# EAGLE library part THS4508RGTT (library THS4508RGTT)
Wideband Fully Differential Amplifier Source: Datasheet
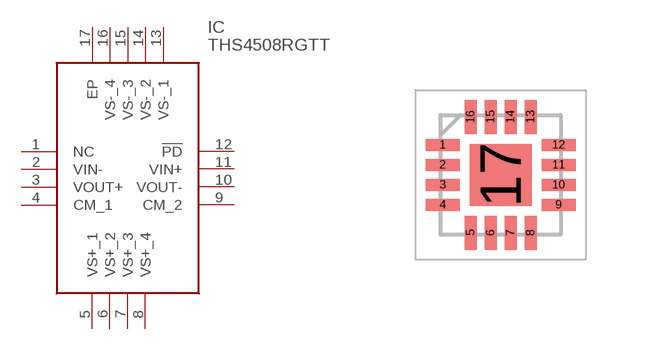
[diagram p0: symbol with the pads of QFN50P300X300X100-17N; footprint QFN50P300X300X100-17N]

Designator prefix IC

## THS4508RGTT (Description: Wideband Fully Differential Amplifier; Height: 1mm; Manufacturer_Name: Texas Instruments; Manufacturer_Part_Number: THS4508RGTT; Mouser_Part_Number: 595-THS4508RGTT; Mouser_Price-Stock: https://www.mouser.co.uk/ProductDetail/Texas-Instruments/THS4508RGTT?qs=ZmJdcv7QZ9qPmiKnIsJUNg%3D%3D)  [QFN50P300X300X100-17N]
1  NC  nc
2  VIN-
3  VOUT+
4  CM_1
5  VS+_1
6  VS+_2
7  VS+_3
8  VS+_4
9  CM_2
10  VOUT-
11  VIN+
12  !PD
13  VS-_1
14  VS-_2
15  VS-_3
16  VS-_4
17  EP

## Footprint QFN50P300X300X100-17N (pad centres in mm)
RGT0016A_2021-1
smd 0.85 x 0.3: 1 -1.45,0.75; 2 -1.45,0.25; 3 -1.45,-0.25; 4 -1.45,-0.75; 9 1.45,-0.75; 10 1.45,-0.25; 11 1.45,0.25; 12 1.45,0.75
smd 0.3 x 0.85: 5 -0.75,-1.45; 6 -0.25,-1.45; 7 0.25,-1.45; 8 0.75,-1.45; 13 0.75,1.45; 14 0.25,1.45; 15 -0.25,1.45; 16 -0.75,1.45
smd 1.55 x 1.55: 17 0,0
